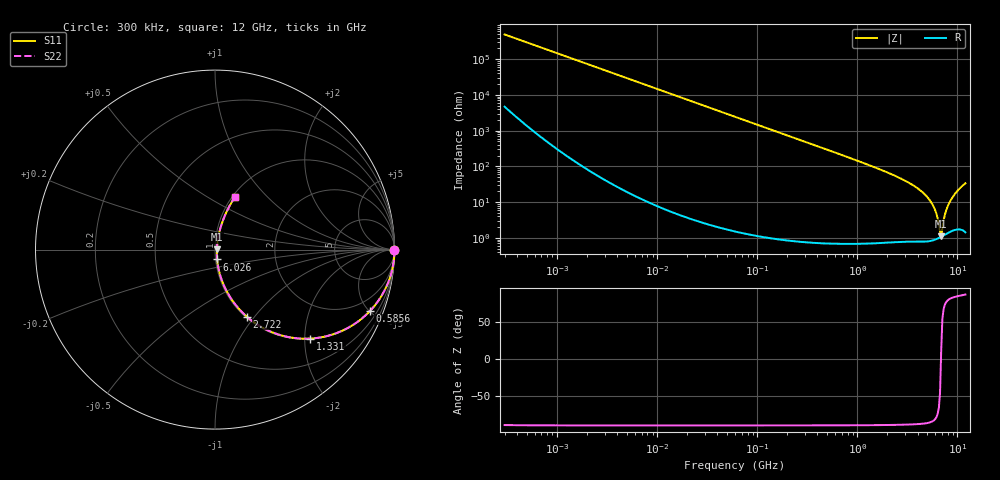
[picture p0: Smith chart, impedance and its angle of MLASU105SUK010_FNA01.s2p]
! MLASU105SUK010_FNA01  S-PARAMETER MODEL  ( General Type )
! Model Generated by TAIYO YUDEN Corporation (http://www.ty-top.com)
! Version 2.0
! TAIYO YUDEN Control No. 120810
! Copyright(c) 2011 TAIYO YUDEN CO.,LTD. All Rights Reserved.
! Product Description (link to TY-COMPAS)
! https://ds.yuden.co.jp/TYCOMPAS/or/detail?pn=MLASU105SUK010CFNA01&u=M
! Products Name : Multilayer Ceramic Capacitors
! Characteristics :
!  Capacitance : 1 pF , Rated Voltage : 50V , TCC : UK / U2K
!  Case Size : 1.0 x 0.5 / 0.039 x 0.02 [mm/inch] , Thickness : 0.5 / 0.02 [mm/inch]
!  (Conditions: Temperature = 25 degC , DC Bias Current/Voltage = 0A / 0V)
! External Node Assignments :
!  1  o---| |---o  2
! GND o---------o GND
! Frequency Range : 0.3MHz  -  12000MHz  [ 401 STEP ]
# MHz S RI R 50
! Freq[MHz].  S11 Real  S11 Imag  S21 Real  S21 Imag  S12 Real  S12 Imag  S22 Real  S22 Imag
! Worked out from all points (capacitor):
!   401 points, 300 kHz to 12 GHz, reference 50 ohm
!   read as one part in series: C = 1.08 pF near 316.3 kHz
!   lowest |Z| = 1.1 ohm at 6.88 GHz (marker M1)
!   series resonance near 6.848 GHz, so ESL is about 500 pH
!   S11 on the Smith chart (normalised r, x): 300 kHz: open; 585.6 MHz: 1.01, -5.00; 1.331 GHz: 1.01, -2.13; 2.722 GHz: 1.02, -0.91; 6.026 GHz: 1.02, -0.11; 12 GHz: 1.03, +0.67
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0.3  1 -0.000203  1.97e-06 0.000203  1.97e-06 0.000203  1 -0.000203
1.769972  1 -0.0012  2.92e-06 0.0012  2.92e-06 0.0012  1 -0.0012
10.44266  0.9999 -0.00708  5.38e-05 0.00708  5.38e-05 0.00708  0.9999 -0.00708
60  0.9983 -0.0406  0.00168 0.0406  0.00168 0.0406  0.9983 -0.0406
159.8975  0.9883 -0.1072  0.0117 0.1072  0.0117 0.1072  0.9883 -0.1072
353.9943  0.9449 -0.2273  0.0551 0.2273  0.0551 0.2273  0.9449 -0.2273
585.5907  0.8614 -0.3441  0.1386 0.3441  0.1386 0.3441  0.8614 -0.3441
871.3074  0.7342 -0.4397  0.2658 0.4397  0.2658 0.4397  0.7342 -0.4397
1331.232  0.5319 -0.4957  0.4681 0.4957  0.4681 0.4957  0.5319 -0.4957
2088.533  0.2934 -0.4495  0.7066 0.4495  0.7066 0.4495  0.2934 -0.4495
2722.03  0.1767 -0.3731  0.8233 0.3731  0.8233 0.3731  0.1767 -0.3731
3642.919  0.0841 -0.2643  0.9159 0.2643  0.9159 0.2643  0.0841 -0.2643
4623.766  0.0366 -0.1666  0.9634 0.1666  0.9634 0.1666  0.0366 -0.1666
5420.343  0.0183 -0.0997  0.9817 0.0997  0.9817 0.0997  0.0183 -0.0997
6026.253  0.012 -0.0549  0.988 0.0549  0.988 0.0549  0.012 -0.0549
6524.734  0.0103 -0.0214  0.9897 0.0214  0.9897 0.0214  0.0103 -0.0214
6879.757  0.0106 0.00219  0.9894 -0.00219  0.9894 -0.00219  0.0106 0.00219
7064.448  0.0113 0.015  0.9887 -0.015  0.9887 -0.015  0.0113 0.015
7854.144  0.0172 0.0643  0.9828 -0.0643  0.9828 -0.0643  0.0172 0.0643
8503.825  0.0257 0.1039  0.9743 -0.1039  0.9743 -0.1039  0.0257 0.1039
9968.853  0.0551 0.19  0.9449 -0.19  0.9449 -0.19  0.0551 0.19
12000  0.1114 0.2941  0.8886 -0.2941  0.8886 -0.2941  0.1114 0.2941
